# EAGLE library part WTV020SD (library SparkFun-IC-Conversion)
WTV020SD Audio Module SD audio playback IC Can play back .wav or .ad4 files from an SD card SPI control or digital input trigger control available in SSOP-20 or DIP-20 Datasheet SparkFun Products SparkFun Audio-Sound Breakout - WTV020SD (WIG-11125)
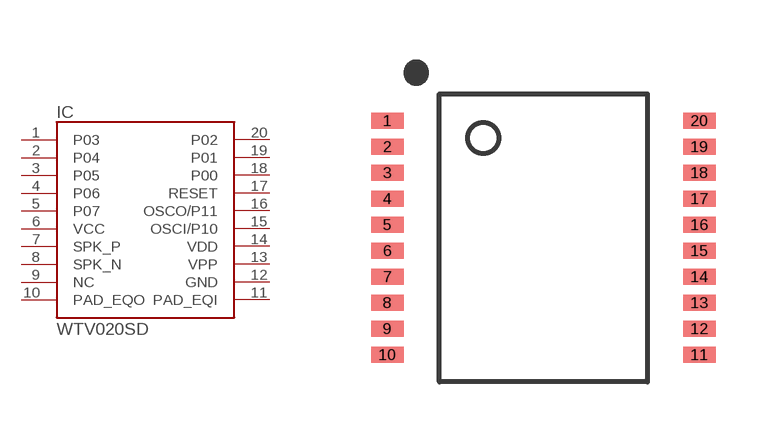
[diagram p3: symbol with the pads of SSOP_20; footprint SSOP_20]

Designator prefix IC

## WTV020SD (PROD_ID: IC-11012; VALUE: WTV020SD-20S)  [SSOP_20]
1  P03
2  P04
3  P05
4  P06
5  P07
6  VCC
7  SPK_P
8  SPK_N
9  NC
10  PAD_EQO
11  PAD_EQI
12  GND
13  VPP
14  VDD
15  OSCI/P10
16  OSCO/P11
17  RESET
18  P00
19  P01
20  P02

## Footprint SSOP_20 (pad centres in mm)
20-pin .65mm pitch/5.2mm body SMT
smd 0.813 x 0.406: 1 -3.9,2.925; 2 -3.9,2.275; 3 -3.9,1.625; 4 -3.9,0.975; 5 -3.9,0.325; 6 -3.9,-0.325; 7 -3.9,-0.975; 8 -3.9,-1.625; 9 -3.9,-2.275; 10 -3.9,-2.925; 11 3.9,-2.925; 12 3.9,-2.275; 13 3.9,-1.625; 14 3.9,-0.975; 15 3.9,-0.325; 16 3.9,0.325; 17 3.9,0.975; 18 3.9,1.625; 19 3.9,2.275; 20 3.9,2.925

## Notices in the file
Licensing: Creative Commons ShareAlike 4.0 International - https://creativecommons.org/licenses/by-sa/4.0
